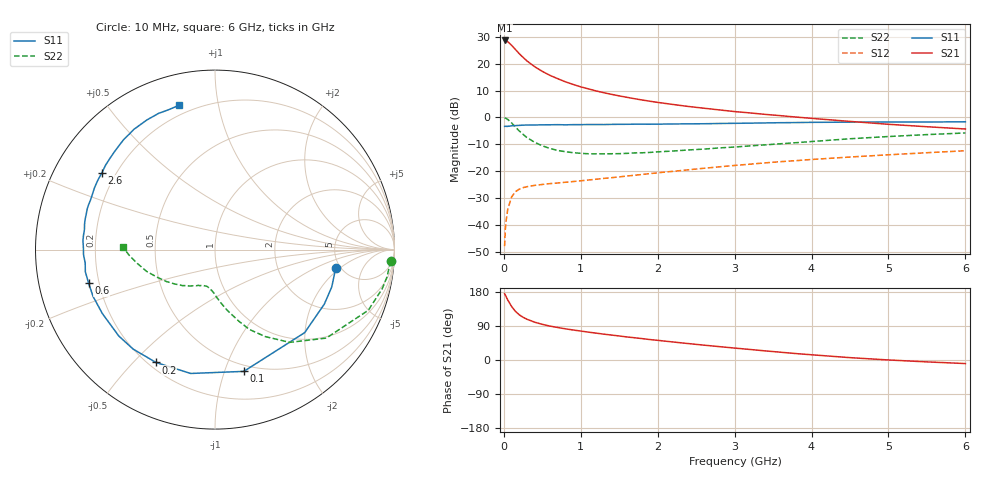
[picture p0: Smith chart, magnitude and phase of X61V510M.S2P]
! SIEMENS Small Signal Semiconductors
! BFP193W
! Si NPN RF Bipolar Junction Transistor in SOT343
! VCE = 1.5 V  IC = 10 mA
! Common Emitter S-Parameters:  April 1994
# GHz  S  MA  R  50
!  f  S11  S21  S12  S22
! GHz  MAG  ANG  MAG  ANG  MAG  ANG  MAG  ANG
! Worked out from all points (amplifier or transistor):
!   40 points, 10 MHz to 6 GHz, reference 50 ohm
!   highest |S21| = 28.7 dB at 10 MHz (marker M1)
!   |S21| within 3 dB of that: start of sweep to 139.3 MHz
!   unconditionally stable (mu >= 1): 1.239 GHz to 4.365 GHz
!   at 200 MHz: K = 0.23, MSG = 25.2 dB, |S12| = -26.7 dB
!   at 1.5 GHz: K = 1.08, MAG = 13.4 dB, |S12| = -22.2 dB
!   at 6 GHz: K = 0.94, MSG = 4.0 dB, |S12| = -12.4 dB
!   S11 on the Smith chart (normalised r, x): 10 MHz: 4.54, -1.76; 100 MHz: 0.44, -1.16; 200 MHz: 0.23, -0.58; 600 MHz: 0.16, -0.13; 2.6 GHz: 0.15, +0.30; 6 GHz: 0.15, +0.77
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0.01  0.6802 -8.8  27.09 174.8  0.004 87.1  0.9805 -3.7
0.02  0.683 -17.7  27.03 171.2  0.0084 82.2  0.9705 -9.0
0.03  0.6806 -26.5  26.74 167.0  0.012 78.8  0.9563 -13.3
0.05  0.6809 -42.8  25.72 158.6  0.0192 71.3  0.9184 -21.6
0.1  0.6972 -76.7  22.1 141.5  0.0328 56.4  0.7921 -38.5
0.15  0.7033 -101.1  18.45 128.4  0.0414 46.5  0.6632 -51.2
0.2  0.7096 -117.6  15.39 119.4  0.046 40.1  0.5595 -60.0
0.25  0.7179 -129.5  13.13 112.7  0.0492 36.0  0.4843 -66.7
0.3  0.7205 -138.1  11.27 107.6  0.0512 33.5  0.4216 -71.5
0.4  0.7218 -150.5  8.809 99.8  0.0542 30.7  0.3442 -78.7
0.5  0.7277 -159.0  7.197 94.1  0.0564 30.3  0.2957 -84.1
0.6  0.7286 -165.2  6.056 89.5  0.0585 30.1  0.2637 -88.3
0.8  0.727 -174.1  4.605 82.3  0.062 32.2  0.2293 -94.3
1.1  0.7373 176.3  3.395 73.5  0.0683 35.5  0.2103 -101.6
1.3  0.7359 171.2  2.879 68.2  0.0731 37.8  0.2097 -105.5
1.6  0.7443 164.5  2.365 60.8  0.0811 40.6  0.2138 -110.9
2.2  0.7547 152.8  1.74 47.5  0.0991 44.3  0.2364 -121.5
2.6  0.7619 145.7  1.483 39.2  0.1128 45.2  0.2567 -128.7
3.2  0.7816 135.8  1.211 27.8  0.1346 44.9  0.2947 -139.4
4.5  0.8159 117.7  0.842 6.2  0.1828 39.8  0.4002 -162.4
5.5  0.8209 108.6  0.67 -5.0  0.2199 34.7  0.4783 -176.1
6  0.8284 104.0  0.608 -9.4  0.2394 32.2  0.513 178.5
